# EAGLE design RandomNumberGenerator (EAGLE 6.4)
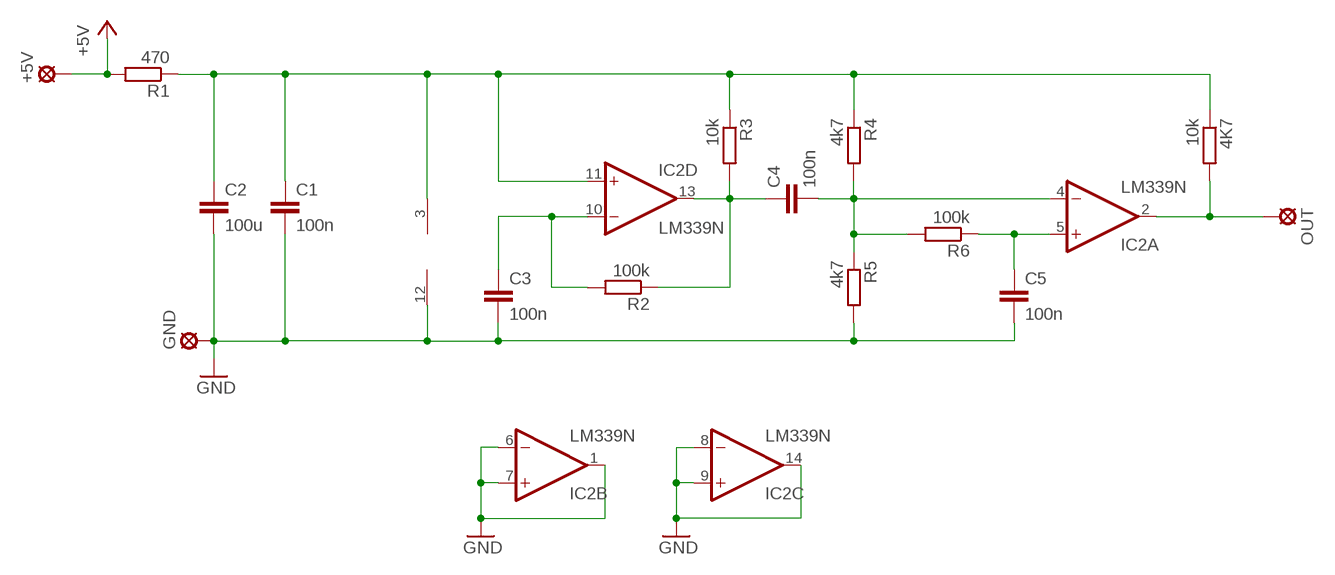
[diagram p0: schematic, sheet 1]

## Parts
4K7  10k  R-EU_0204/2V  [0204V]
+5V  LSP10  [LSP10]
C1  100n  C-EU025-030X050  [C025-030X050]
C2  100u  C-EU102-054X133  [C102-054X133]
C3  100n  C-EU050-025X075  [C050-025X075]
C4  100n  C-EU050-025X075  [C050-025X075]
C5  100n  C-EU050-025X075  [C050-025X075]
GND  LSP10  [LSP10]
IC2  LM339N  [DIL14]
OUT  LSP10  [LSP10]
R1  470  R-EU_0204/7  [0204/7]
R2  100k  R-EU_0204/7  [0204/7]
R3  10k  R-EU_0309/10  [0309/10]
R4  4k7  R-EU_0204/2V  [0204V]
R5  4k7  R-EU_0204/5  [0204/5]
R6  100k  R-EU_0204/2V  [0204V]

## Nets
+5V: +5V.MP R1.2
GND: C1.2 C2.2 C3.2 C5.2 GND.MP IC2.1(B:OUT) IC2.6(B:-IN) IC2.7(B:+IN) IC2.8(C:-IN) IC2.9(C:+IN) IC2.12(P:GND) IC2.14(C:OUT) R5.2
N$1: 4K7.1 C1.1 C2.1 IC2.3(P:V+) IC2.11(D:+IN) R1.1 R3.1 R4.1
N$2: C3.1 IC2.10(D:-IN) R2.2
N$3: C4.1 IC2.13(D:OUT) R2.1 R3.2
N$4: C5.1 IC2.5(A:+IN) R6.1
N$6: C4.2 IC2.4(A:-IN) R4.2 R5.1 R6.2
N$14: 4K7.2 IC2.2(A:OUT) OUT.MP

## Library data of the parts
4K7 R1-R6 = rcl:R-EU_: RESISTOR, European symbol
+5V GND OUT = solpad:LSP10: SOLDER PAD
C1-C5 = rcl:C-EU: CAPACITOR, European symbol
IC2 = linear:LM339: Low Power Low Offset Voltage Quad Comparators with open collector; LM139/LM239/LM339/LM2901/LM3302

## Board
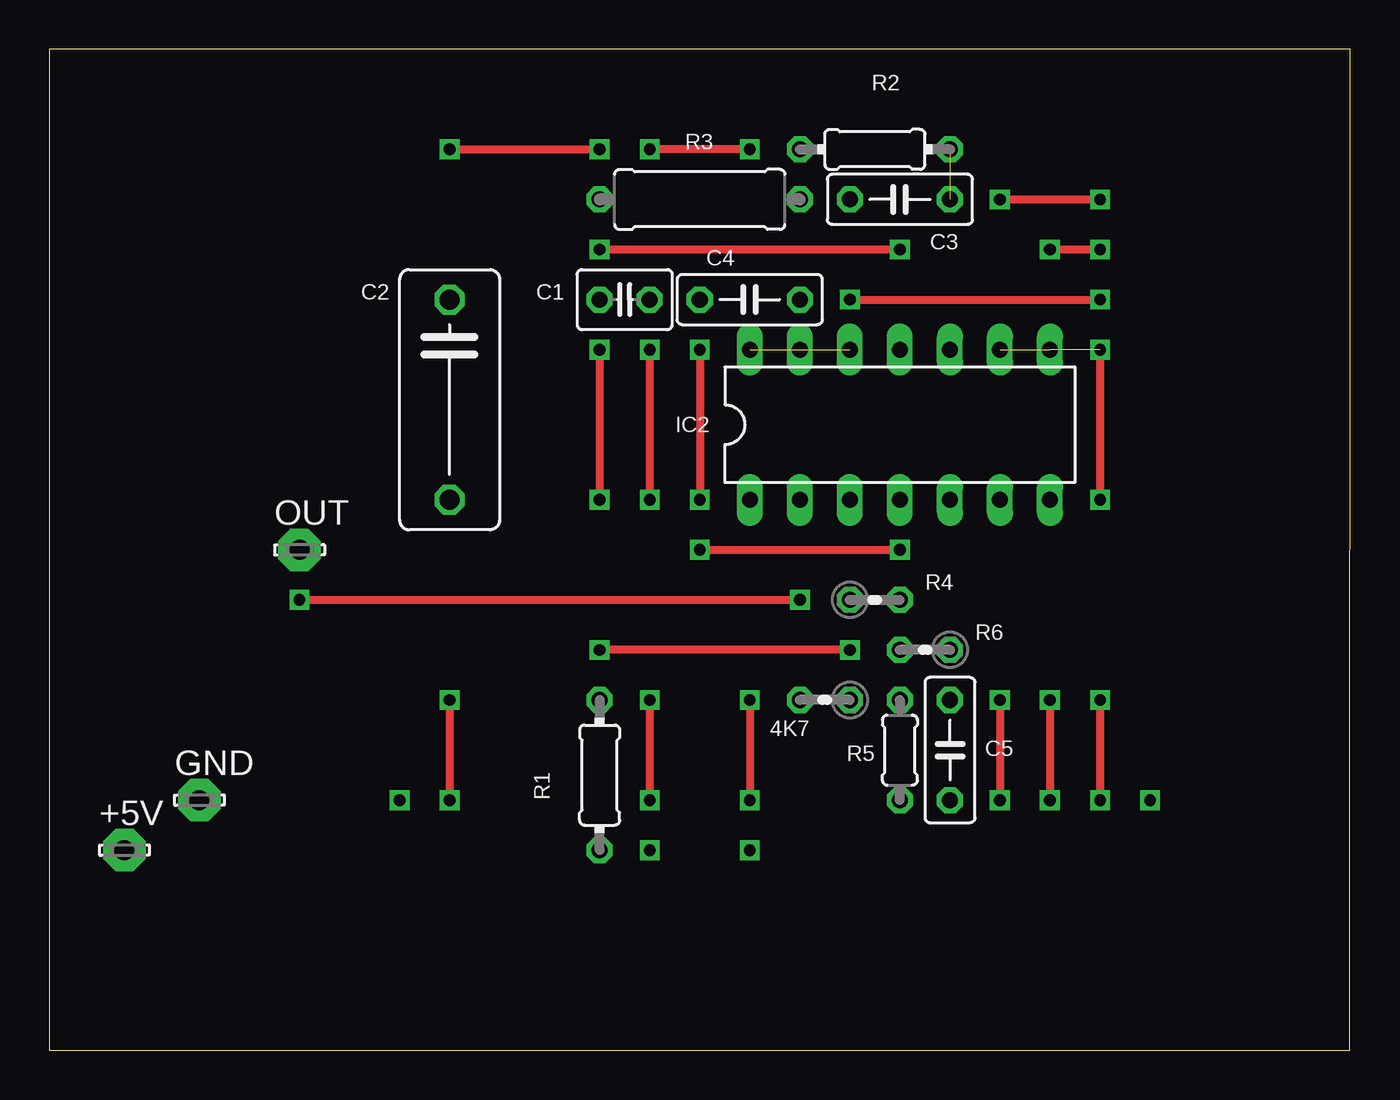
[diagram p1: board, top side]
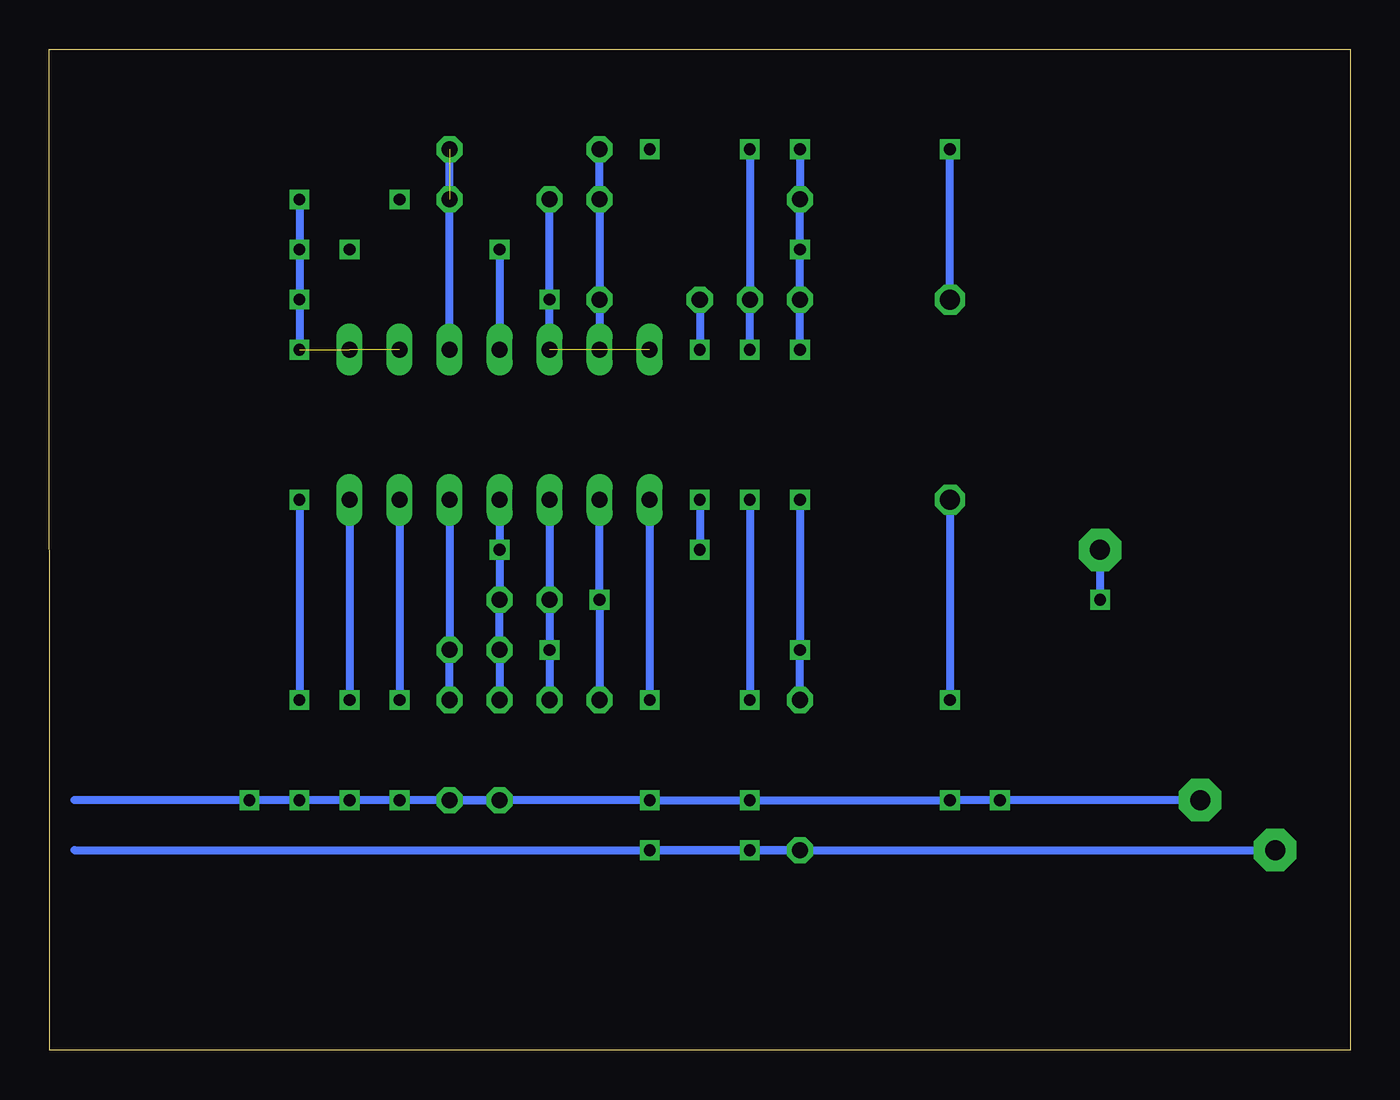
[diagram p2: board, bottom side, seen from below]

Size 66.04 x 50.8 mm. Coordinates in mm from the lower left corner, seen from the top.
Outline: 0,0 66.02,0 66.04,50.8 0,50.8 0,0
Copper layers (1*16): Top 0.035mm / dielectric 1.5mm / Bottom 0.035mm
Design rules "default *": minimum track width 10mil, minimum drill 16mil, track to track 8mil, track to pad 8mil, pad to pad 8mil, via to via 8mil, smd to smd 8mil, copper to edge 40mil, drill to drill 8mil, minimum pad ring 10mil, minimum via ring 8mil, stop-mask expansion 4mil, vias tented up to drill 0mil, thermal gap 10mil

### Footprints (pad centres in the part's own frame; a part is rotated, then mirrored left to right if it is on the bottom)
0204V = drill 0.813 octagon: 1 -1.27,0; 2 1.27,0
LSP10 = drill 1.016 pad 2.159 octagon: MP 0,0
C025-030X050 = drill 0.813 octagon: 1 -1.27,0; 2 1.27,0
C102-054X133 = drill 1.016 octagon: 1 -5.08,0; 2 5.08,0
C050-025X075 = drill 0.813 octagon: 1 -2.54,0; 2 2.54,0
DIL14 = drill 0.813 long: 1 -7.62,-3.81; 2 -5.08,-3.81; 3 -2.54,-3.81; 4 0,-3.81; 5 2.54,-3.81; 6 5.08,-3.81; 7 7.62,-3.81; 8 7.62,3.81; 9 5.08,3.81; 10 2.54,3.81; 11 0,3.81; 12 -2.54,3.81; 13 -5.08,3.81; 14 -7.62,3.81
0204/7 = drill 0.813 octagon: 1 -3.81,0; 2 3.81,0
0309/10 = drill 0.813 octagon: 1 -5.08,0; 2 5.08,0
0204/5 = drill 0.813 octagon: 1 -2.54,0; 2 2.54,0

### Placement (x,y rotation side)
4K7  39.37,17.78 180 top
+5V  3.81,10.16 0 top
C1  29.21,38.1 0 top
C2  20.32,33.02 270 top
C3  43.18,43.18 180 top
C4  35.56,38.1 180 top
C5  45.72,15.24 270 top
GND  7.62,12.7 0 top
IC2  43.18,31.75 0 top
OUT  12.7,25.4 0 top
R1  27.94,13.97 270 top
R2  41.91,45.72 0 top
R3  33.02,43.18 0 top
R4  41.91,22.86 0 top
R5  43.18,15.24 270 top
R6  44.45,20.32 180 top

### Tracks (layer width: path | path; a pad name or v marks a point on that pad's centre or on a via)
+5V  (via drill 0.6)
  Bottom 0.406: 64.77,10.16 R1.2 | R1.2 v35.56,10.16 v30.48,10.16 R1.2 | R1.2 +5V.MP
GND  (via drill 0.6)  (3 unrouted)
  Top 0.406: v40.64,38.1 v53.34,38.1 | v30.48,35.56 v30.48,27.94 | v30.48,17.78 v30.48,12.7 | v53.34,35.56 v53.34,27.94 | v53.34,17.78 v53.34,12.7 | v35.56,17.78 v35.56,12.7 | v50.8,17.78 v50.8,12.7 | v48.26,17.78 v48.26,12.7 | v50.8,40.64 v53.34,40.64 | v48.26,43.18 v53.34,43.18 | v35.56,45.72 v30.48,45.72 | v20.32,17.78 v20.32,12.7
  Bottom 0.406: C5.2 v53.34,12.7 | C5.2 R5.2 | C3.2 v40.64,38.1 IC2.12 | v53.34,35.56 v53.34,38.1 v53.34,40.64 v53.34,43.18 | v53.34,12.7 64.77,12.7 | v30.48,27.94 v30.48,17.78 | v53.34,27.94 v53.34,17.78 | GND.MP v17.78,12.7 v20.32,12.7 v30.48,12.7 v35.56,12.7 v53.34,12.7 | IC2.1 v35.56,17.78 | v53.34,12.7 v55.88,12.7 | C5.2 v48.26,12.7 v50.8,12.7 v53.34,12.7 | IC2.7 v50.8,17.78 | IC2.6 v48.26,17.78 | v30.48,45.72 C1.2 v30.48,35.56 | C2.2 v20.32,17.78
N$1  (via drill 0.6)
  Top 0.406: v27.94,40.64 v43.18,40.64 | v40.64,20.32 v27.94,20.32 | v27.94,35.56 v27.94,27.94 | v20.32,45.72 v27.94,45.72
  Bottom 0.406: 4K7.1 v40.64,20.32 R4.1 IC2.3 | v43.18,40.64 IC2.11 | v27.94,27.94 v27.94,20.32 R1.1 | C2.1 v20.32,45.72 | v27.94,45.72 R3.1 v27.94,40.64 C1.1 v27.94,35.56
N$2  (1 unrouted)
  Bottom 0.406: IC2.10 R2.2
N$3
  Bottom 0.406: IC2.13 C4.1 R3.2 R2.1
N$4
  Bottom 0.406: C5.1 R6.1 IC2.5
N$6  (via drill 0.6)
  Top 0.406: v33.02,35.56 v33.02,27.94 | v33.02,25.4 v43.18,25.4
  Bottom 0.406: C4.2 v33.02,35.56 | v33.02,27.94 v33.02,25.4 | IC2.4 v43.18,25.4 R4.2 R6.2 R5.1
N$14  (via drill 0.6)
  Top 0.406: v12.7,22.86 v38.1,22.86
  Bottom 0.406: IC2.2 v38.1,22.86 4K7.2 | OUT.MP v12.7,22.86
